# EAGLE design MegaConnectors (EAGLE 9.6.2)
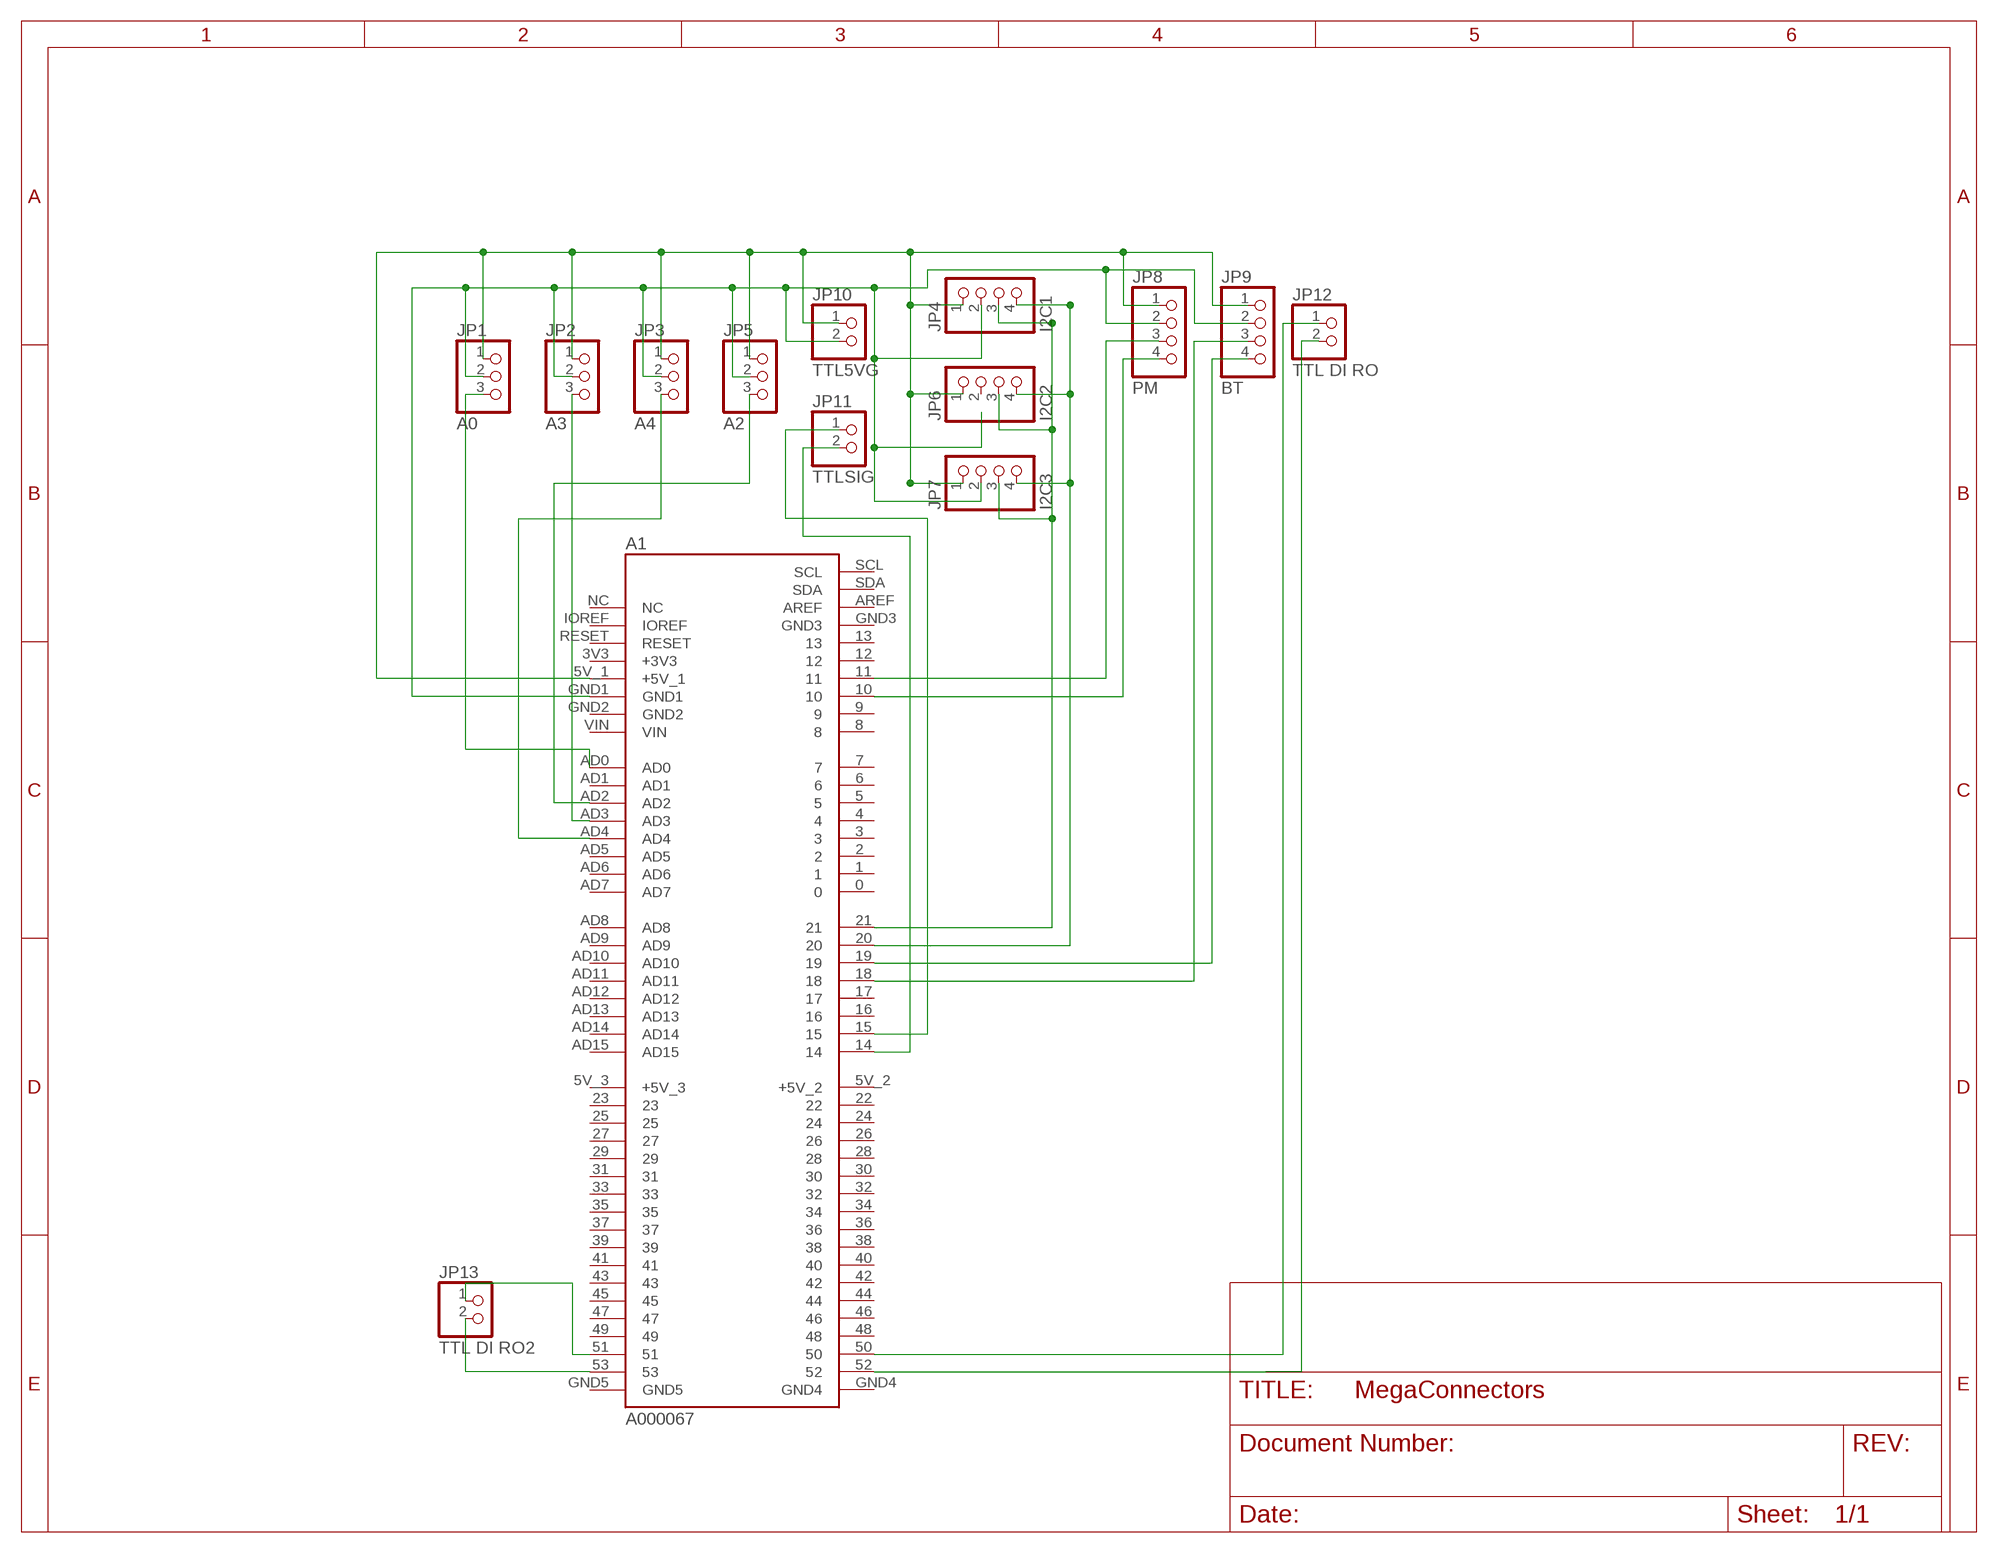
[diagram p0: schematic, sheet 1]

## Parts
A1  A000067  [ARDUINO_A000067]
JP1  A0  PINHD-1X3  [1X03]
JP2  A3  PINHD-1X3  [1X03]
JP3  A4  PINHD-1X3  [1X03]
JP4  I2C1  PINHD-1X4  [1X04]
JP5  A2  PINHD-1X3  [1X03]
JP6  I2C2  PINHD-1X4  [1X04]
JP7  I2C3  PINHD-1X4  [1X04]
JP8  PM  PINHD-1X4  [1X04]
JP9  BT  PINHD-1X4  [1X04]
JP10  TTL5VG  PINHD-1X2  [1X02]
JP11  TTLSIG  PINHD-1X2  [1X02]
JP12  TTL DI RO  PINHD-1X2  [1X02]
JP13  TTL DI RO2  PINHD-1X2  [1X02]

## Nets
N$1: A1.5V_1(+5V_1) JP1.1 JP2.1 JP3.1 JP4.1 JP5.1 JP6.1 JP7.1 JP8.1 JP9.1 JP10.1
N$2: A1.GND1 JP1.2 JP2.2 JP3.2 JP4.2 JP5.2 JP7.2 JP8.2 JP9.2 JP10.2
N$3: A1.AD0 JP1.3
N$4: A1.AD2 JP5.3
N$5: A1.AD3 JP2.3
N$6: A1.AD4 JP3.3
N$7: A1.18 JP9.3
N$8: A1.11 JP8.3
N$9: A1.20 JP4.4 JP6.4 JP7.4
N$10: A1.21 JP4.3 JP6.3 JP7.3
N$11: A1.10 JP8.4
N$12: A1.19 JP9.4
N$13: A1.50 JP12.1
N$14: A1.15 JP11.1
N$15: A1.14 JP11.2
N$16: A1.52 JP12.2
N$17: A1.51 JP13.1
N$18: A1.53 JP13.2
Unconnected: A1.0 A1.1 A1.2 A1.3 A1.3V3(+3V3) A1.4 A1.5 A1.5V_2(+5V_2) A1.5V_3(+5V_3) A1.6 A1.7 A1.8 A1.9 A1.12 A1.13 A1.16 A1.17 A1.22 A1.23 A1.24 A1.25 A1.26 A1.27 A1.28 A1.29 A1.30 A1.31 A1.32 A1.33 A1.34 A1.35 A1.36 A1.37 A1.38 A1.39 A1.40 A1.41 A1.42 A1.43 A1.44 A1.45 A1.46 A1.47 A1.48 A1.49 A1.AD1 A1.AD5 A1.AD6 A1.AD7 A1.AD8 A1.AD9 A1.AD10 A1.AD11 A1.AD12 A1.AD13 A1.AD14 A1.AD15 A1.AREF A1.GND2 A1.GND3 A1.GND4 A1.GND5 A1.IOREF A1.NC A1.RESET A1.SCL A1.SDA A1.VIN JP6.2

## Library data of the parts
A1 = mega2560:A000067: ARDUINO UNO REV3 DEVELOPMENT BOARD; DESCRIPTION: Arduino Mega 2560 Rev3. ATmega2560 Microcontroller Mega Development Board 16MHz CPU 8KB RAM 4KB/256KB EEPROM/Flash; DIGI-KEY_PART_NUMBER: 1050-1018-ND; MF: Arduino; MP: A000067; PACKAGE: Non-Standard Arduino; PURCHASE-URL: https://pricing.snapeda.com/search/part/A000067/?ref=eda
JP1-JP3 JP5 = pinhead:PINHD-1X3: PIN HEADER
JP4 JP6-JP9 = pinhead:PINHD-1X4: PIN HEADER
JP10-JP13 = pinhead:PINHD-1X2: PIN HEADER

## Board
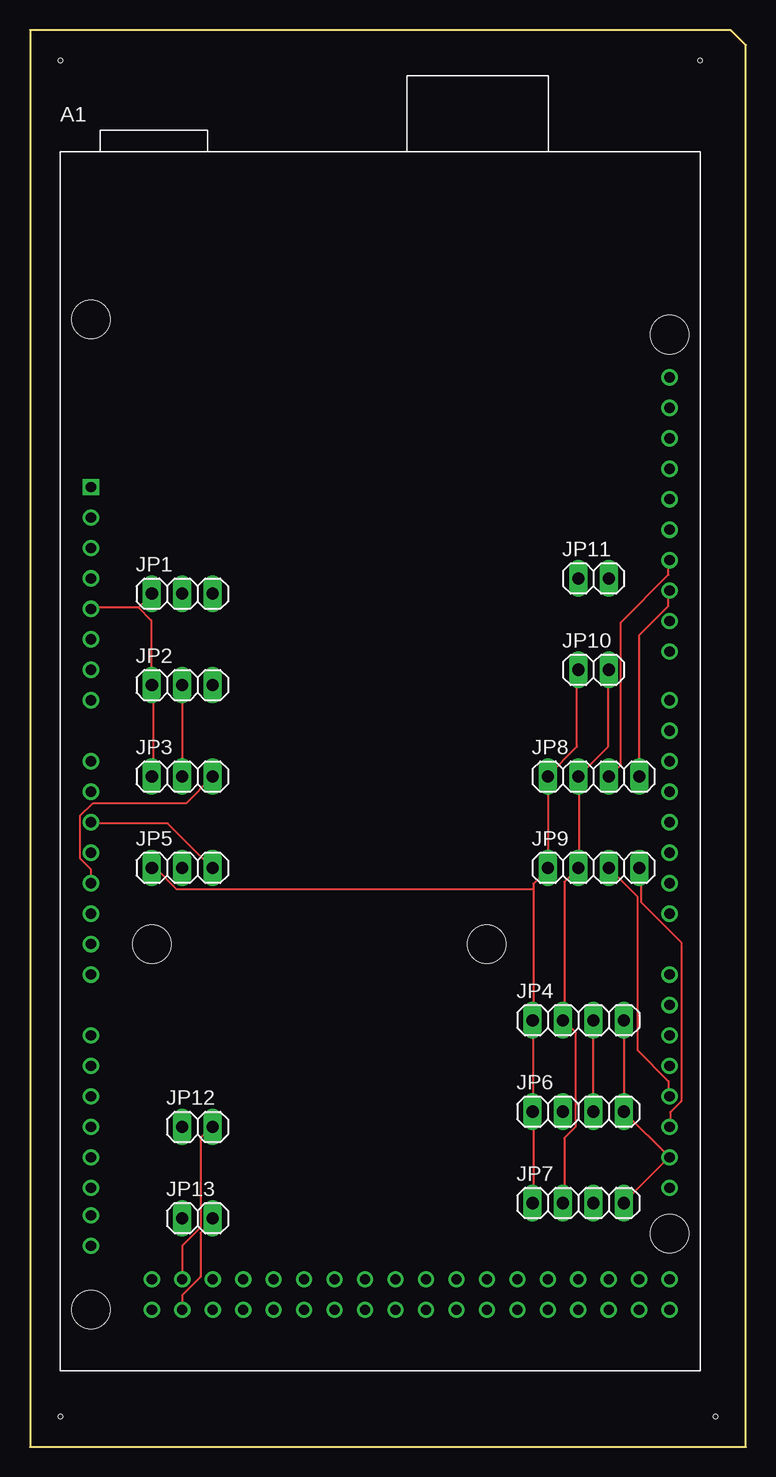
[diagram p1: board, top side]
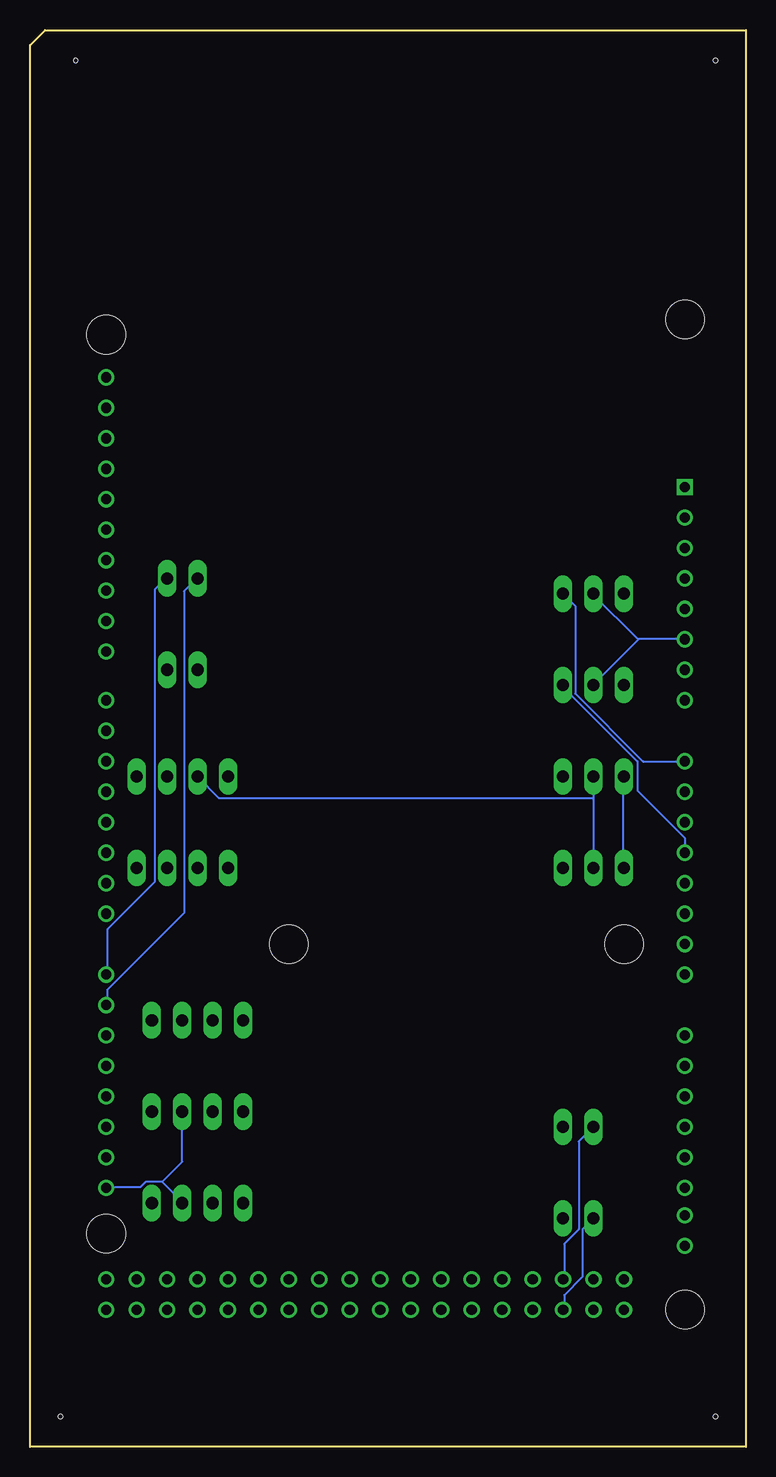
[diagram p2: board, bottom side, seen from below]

Size 59.69 x 118.11 mm. Coordinates in mm from the lower left corner, seen from the top.
Outline: 58.42,118.11 0,118.11 0,0 59.69,0 59.69,116.84 58.42,118.11
Copper layers (1*16): Top 0.035mm / dielectric 1.5mm / Bottom 0.035mm
Design rules "default": minimum track width 6mil, minimum drill 0.35mm, track to track 6mil, track to pad 6mil, pad to pad 6mil, via to via 6mil, smd to smd 6mil, copper to edge 40mil, drill to drill 6mil, minimum pad ring 10mil, minimum via ring 8mil, stop-mask expansion 4mil, vias tented up to drill 0mil, thermal gap 10mil
Holes 0.35 mm at 2.54,115.57 55.88,115.57 2.54,2.54 57.15,2.54

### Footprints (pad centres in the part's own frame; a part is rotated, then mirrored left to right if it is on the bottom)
ARDUINO_A000067 = drill 0.85: 0 24.13,-12.7; 1 24.13,-10.16; 2 24.13,-7.62; 3 24.13,-5.08; 3V3 -24.13,15.24; 4 24.13,-2.54; 5 24.13,0; 5V_1 -24.13,12.7; 5V_2 24.13,-43.18; 5V_3 24.13,-45.72; 6 24.13,2.54; 7 24.13,5.08; 8 24.13,9.144; 9 24.13,11.684; 10 24.13,14.224; 11 24.13,16.764; 12 24.13,19.304; 13 24.13,21.844; 14 24.13,-17.78; 15 24.13,-20.32; 16 24.13,-22.86; 17 24.13,-25.4; 18 24.13,-27.94; 19 24.13,-30.48; 20 24.13,-33.02; 21 24.13,-35.56; 22 21.59,-43.18; 23 21.59,-45.72; 24 19.05,-43.18; 25 19.05,-45.72; 26 16.51,-43.18; 27 16.51,-45.72; 28 13.97,-43.18; 29 13.97,-45.72; 30 11.43,-43.18; 31 11.43,-45.72; 32 8.89,-43.18; 33 8.89,-45.72; 34 6.35,-43.18; 35 6.35,-45.72; 36 3.81,-43.18; 37 3.81,-45.72; 38 1.27,-43.18; 39 1.27,-45.72; 40 -1.27,-43.18; 41 -1.27,-45.72; 42 -3.81,-43.18; 43 -3.81,-45.72; 44 -6.35,-43.18; 45 -6.35,-45.72; 46 -8.89,-43.18; 47 -8.89,-45.72; 48 -11.43,-43.18; 49 -11.43,-45.72; 50 -13.97,-43.18; 51 -13.97,-45.72; 52 -16.51,-43.18; 53 -16.51,-45.72; AD0 -24.13,0; AD1 -24.13,-2.54; AD2 -24.13,-5.08; AD3 -24.13,-7.62; AD4 -24.13,-10.16; AD5 -24.13,-12.7; AD6 -24.13,-15.24; AD7 -24.13,-17.78; AD8 -24.13,-22.86; AD9 -24.13,-25.4; AD10 -24.13,-27.94; AD11 -24.13,-30.48; AD12 -24.13,-33.02; AD13 -24.13,-35.56; AD14 -24.13,-37.846; AD15 -24.13,-40.386; AREF 24.13,26.924; GND1 -24.13,10.16; GND2 -24.13,7.62; GND3 24.13,24.384; GND4 -19.05,-43.18; GND5 -19.05,-45.72; IOREF -24.13,20.32; RESET -24.13,17.78; SCL 24.13,32.004; SDA 24.13,29.464; VIN -24.13,5.08 | drill 0.85 square: NC -24.13,22.86 | hole 3.2: -24.13,36.83; -19.05,-15.24; 8.89,-15.24; 24.13,35.56; -24.13,-45.72; 24.13,-39.37
1X03 = drill 1.016 long: 1 -2.54,0; 2 0,0; 3 2.54,0
1X04 = drill 1.016 long: 1 -3.81,0; 2 -1.27,0; 3 1.27,0; 4 3.81,0
1X02 = drill 1.016 long: 1 -1.27,0; 2 1.27,0

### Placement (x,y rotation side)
A1  29.21,57.15 0 top
JP1  12.7,71.12 0 top
JP2  12.7,63.5 0 top
JP3  12.7,55.88 0 top
JP4  45.72,35.56 0 top
JP5  12.7,48.26 0 top
JP6  45.72,27.94 0 top
JP7  45.72,20.32 0 top
JP8  46.99,55.88 0 top
JP9  46.99,48.26 0 top
JP10  46.99,64.77 0 top
JP11  46.99,72.39 0 top
JP12  13.97,26.67 0 top
JP13  13.97,19.05 0 top

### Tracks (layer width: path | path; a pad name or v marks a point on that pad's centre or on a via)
N$1
  Top 0.152: 9.04,69.95 5.08,69.95 A1.5V_1 | 9.04,69.95 10.11,71.02 JP1.1 | 9.04,69.95 10.11,68.89 10.11,63.55 JP2.1 10.26,63.4 10.26,55.93 JP3.1 | JP7.1 41.96,20.42 41.96,27.89 JP6.1 41.96,28.04 41.96,35.51 JP4.1 41.96,35.66 41.96,46.48 | JP10.1 45.62,64.77 45.62,58.37 43.18,55.93 JP8.1 JP9.1 43.18,48.16 41.96,46.94 41.96,46.48 | 41.96,46.48 12.24,46.48 10.57,48.16 10.26,48.16 JP5.1
  Bottom 0.152: JP5.1 10.26,48.31 10.26,55.78 JP3.1
N$2
  Top 0.152: JP2.2 JP3.2 | JP7.2 44.55,20.42 44.55,25.76 45.47,26.67 45.47,34.59 44.55,35.51 JP4.2 44.55,35.66 44.55,47.09 JP9.2 45.77,48.31 45.77,55.78 JP8.2 48.21,58.37 48.21,64.77 JP10.2
  Bottom 0.152: JP3.2 12.7,54.1 | 12.7,54.1 JP5.2 | 8.89,67.36 9.04,67.36 12.7,71.02 JP1.2 | 8.89,67.36 5.08,67.36 A1.GND1 | 8.89,67.36 12.7,63.55 JP2.2 | 12.7,54.1 43.94,54.1 JP8.2
N$3
  Bottom 0.152: A1.AD0 8.58,57.15 14.22,62.79 14.22,70.1 JP1.3
N$4
  Top 0.152: A1.AD2 5.08,51.97 11.48,51.97 15.14,48.31 JP5.3
N$5
  Bottom 0.152: A1.AD3 5.08,50.75 9.04,54.71 9.04,57.15 15.29,63.4 JP2.3
N$6
  Top 0.152: A1.AD4 5.08,48.16 4.17,49.07 4.17,52.58 5.23,53.65 13,53.65 JP3.3
N$7
  Top 0.152: JP9.3 50.65,45.87 50.65,33.07 53.24,30.48 53.24,29.26 A1.18
N$8
  Top 0.152: A1.11 53.24,73.91 53.24,72.7 49.28,68.73 49.28,56.84 48.36,55.93 JP8.3
N$9
  Top 0.152: JP7.4 49.58,20.42 53.24,24.08 A1.20 JP6.4 49.58,28.04 49.58,35.51 JP4.4
N$10
  Top 0.152: JP6.3 JP4.3
  Bottom 0.152: 48.67,22.1 50.04,22.1 50.49,21.64 53.24,21.64 A1.21 | 48.67,22.1 46.99,20.42 JP7.3 | JP6.3 46.99,23.77 48.67,22.1
N$11
  Top 0.152: JP8.4 50.8,67.67 53.24,70.1 53.24,71.32 A1.10
N$12
  Top 0.152: A1.19 53.39,26.67 53.39,27.89 54.3,28.8 54.3,42.06 50.95,45.41 50.95,48.01 50.8,48.16 JP9.4
N$13
  Bottom 0.152: JP12.1 13.92,25.45 13.92,18.14 15.14,16.92 15.14,14.02 A1.50
N$14
  Bottom 0.152: A1.15 53.24,36.88 53.24,38.1 46.84,44.5 46.84,71.32 45.77,72.39 JP11.1
N$15
  Bottom 0.152: A1.14 53.24,39.47 53.24,43.13 49.28,47.09 49.28,71.48 48.36,72.39 JP11.2
N$16
  Top 0.152: A1.52 12.7,16.76 14.22,18.29 14.22,25.76 15.14,26.67 JP12.2
N$17
  Bottom 0.152: JP13.1 13.61,18.14 13.61,14.17 15.14,12.65 15.14,11.43 A1.51
N$18
  Top 0.152: A1.53 12.7,12.65 14.22,14.17 14.22,17.83 15.14,18.75 15.14,19.05 JP13.2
